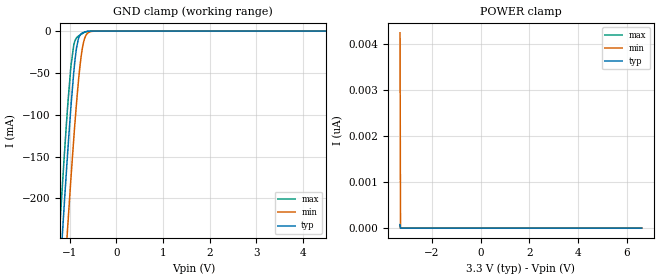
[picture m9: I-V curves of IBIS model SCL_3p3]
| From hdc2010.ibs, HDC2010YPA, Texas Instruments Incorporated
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[Model]   SCL_3p3
Model_type   Input
Vinl = 0.99
Vinh = 2.31
|   typ   min   max
|   (nom PVT)   (slow PVT)   (fast PVT)
C_comp   0.655p   0.636p   0.670p
[Model spec]
|subparameter
Vinl   0.99   0.90   1.08
Vinh   2.31   2.10   2.52
[Voltage Range]   3.3   3   3.6
[Temperature Range]   27   125   -40
[Power Clamp Reference]   3.3   3   3.6
[GND Clamp Reference]   0   0   0
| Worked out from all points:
|   GND clamp passes 1 mA (typ) near -0.68 V on its own axis
[GND Clamp]
|   Voltage   I(typ)   I(min)   I(max)
-3.3V     -2.315A    -2.395A    -2.265A
-1.221V   -298.7mA   -389.7mA   -240.1mA
-1.122V   -210.6mA   -301.2mA   -152.7mA
-1.053V   -151.6mA   -241mA     -95.72mA
-973.5mV  -89.1mA    -174.9mA   -41.13mA
-884.4mV  -32.64mA   -106.2mA   -10.96mA
-815.1mV  -9.285mA   -60.38mA   -5.908mA
-755.7mV  -3.293mA   -30.16mA   -3.85mA
-706.2mV  -1.606mA   -13.9mA    -2.17mA
-627mV    -422.5uA   -3.004mA   -488.3uA
-468.6mV  -9.411uA   -107.7uA   -3.259uA
6.6V      0A         0A         0A
[POWER Clamp]
|   Voltage   I(typ)   I(min)   I(max)
-3.3V     78.12pA    4.245nA    62.09pA
-3.28V    0A         0A         0A
-3.27V    0A         0A         0A
6.6V      0A         0A         0A
